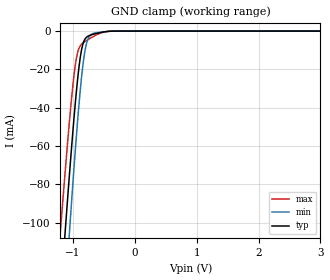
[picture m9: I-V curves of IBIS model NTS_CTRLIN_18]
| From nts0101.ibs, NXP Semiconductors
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|   Model NTS_CTRLIN_18
[Model]   NTS_CTRLIN_18
Model_type   Input
Vinh  =  1.170 | 0.65*Vcc
Vinl  =  0.630 | 0.35*Vcc
C_comp   0.7044pF   0.5503pF   0.9953pF
[Model Spec]
| Note: The input and output voltage ratings may be exceeded if the input and
|   output current ratings are observed (please refer to the data sheet)
|   Subparameter   typ   min   max
Vinh   1.170   1.073   1.268
Vinl   0.630   0.578   0.683
| Overshoot
S_overshoot_high   6.5   6.5   6.5   | Static overshoot
S_overshoot_low   -0.5   -0.5   -0.5
D_overshoot_high   7.2   7.2   7.2   | Dynamic overshoot
D_overshoot_low   -1.0   -1.0   -1.0
D_overshoot_time   3n   3n   3n
|Ambient temperature:   25   85   -40
[Temperature Range]   35   95   -35
[Voltage Range]   1.8   1.65   1.95
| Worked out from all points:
|   GND clamp passes 1 mA (typ) near -0.58 V on its own axis
|Process Range   nominal   slow   fast
[GND_clamp]
|   voltage   I(typ)   I(min)   I(max)
-5.5V     -2.243A    -2.508A    -2.023A
-1.2V     -138.9mA   -176.6mA   -104.2mA
-1.12V    -103mA     -136.7mA   -71.92mA
-1.06V    -77.14mA   -107.7mA   -49.04mA
-1.04V    -68.78mA   -98.29mA   -41.85mA
-960mV    -37.6mA    -62.23mA   -17.76mA
-920mV    -24.3mA    -45.71mA   -10.81mA
-860mV    -9.903mA   -24.3mA    -6.894mA
-780mV    -3.231mA   -6.594mA   -4.942mA
-660mV    -1.583mA   -1.146mA   -2.68mA
-340mV    -20.37uA   -28.22uA   -16.89uA
5.5V      0A         0A         0A
